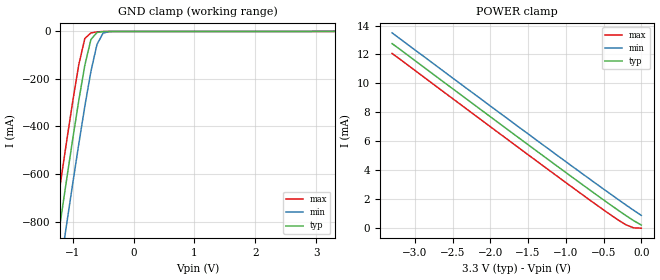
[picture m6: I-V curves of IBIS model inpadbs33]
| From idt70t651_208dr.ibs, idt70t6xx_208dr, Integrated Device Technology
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|   Model inpadbs33
[Model]   inpadbs33
Model_type   Input
Polarity   Non-Inverting
Vinl =  0.80000V
Vinh =  2.00000V
Vmeas =  1.50000V
C_comp   4.50000pF   4.50000pF   4.50000pF
[Temperature Range]   25.00000   100.00000   -40.00000
[Voltage Range]   3.30000V   3.10000V   3.50000V
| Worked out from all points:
|   GND clamp passes 1 mA (typ) near -0.51 V on its own axis
|   POWER clamp passes 1 mA (typ) near -0.24 V on its own axis
[GND_clamp]
| voltage   I(typ)   I(min)   I(max)
-3.3V     -4.611A    -4.788A    -4.461A
-1.4V     -1.152A    -1.34A     -992.6mA
-1.3V     -975mA     -1.163A    -814.6mA
-1.2V     -799.1mA   -987.7mA   -638.4mA
-1.1V     -625.5mA   -813.9mA   -465mA
-900mV    -292mA     -475.5mA   -141.4mA
-800mV    -142.5mA   -315.2mA   -29.67mA
-700mV    -33.98mA   -168.4mA   -6.426mA
-600mV    -4.297mA   -54.25mA   -1.776mA
-500mV    -774.3uA   -6.916mA   -201.4uA
-400mV    -82.6uA    -641.8uA   -19.34uA
3.3V      224.6uA    1.601mA    8.09uA
[POWER_clamp]
| voltage   I(typ)   I(min)   I(max)
-3.3V     12.75mA    13.49mA    12.07mA
-1.3V     5.006mA    5.753mA    4.313mA
-500mV    1.963mA    2.711mA    1.273mA
-200mV    868.8uA    1.601mA    233.9uA
-100mV    528.1uA    1.241mA    32.77uA
0V        224.6uA    891.2uA    11.77uA
